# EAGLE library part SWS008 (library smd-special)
SMD Dip Switch 8 pol.
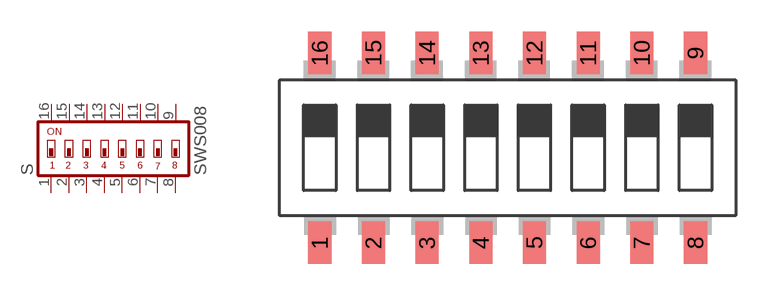
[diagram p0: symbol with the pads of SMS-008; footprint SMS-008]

Designator prefix S

## SWS008  [SMS-008]
1  1  pas
2  2  pas
3  3  pas
4  4  pas
5  5  pas
6  6  pas
7  7  pas
8  8  pas
9  9  pas
10  10  pas
11  11  pas
12  12  pas
13  13  pas
14  14  pas
15  15  pas
16  16  pas

## Footprint SMS-008 (pad centres in mm)
DIP SWITCH
smd 1.092 x 2.007: 1 -8.89,-4.496; 2 -6.35,-4.496; 3 -3.81,-4.496; 4 -1.27,-4.496; 5 1.27,-4.496; 6 3.81,-4.496; 7 6.35,-4.496; 8 8.89,-4.496; 9 8.89,4.496; 10 6.35,4.496; 11 3.81,4.496; 12 1.27,4.496; 13 -1.27,4.496; 14 -3.81,4.496; 15 -6.35,4.496; 16 -8.89,4.496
